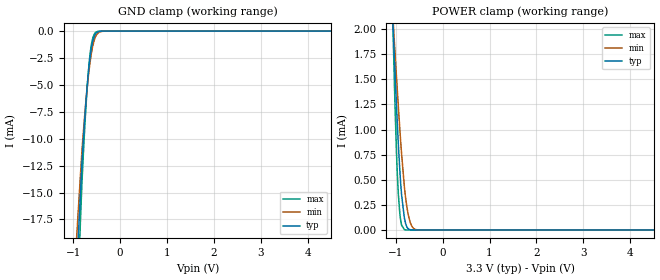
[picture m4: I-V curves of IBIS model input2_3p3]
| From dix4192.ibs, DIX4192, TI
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|   input2_3p3 Model
[Model]   input2_3p3
Model_type   Input
Vinl = 0.99
Vinh = 2.31
|   typ   min   max
C_comp   30.3138pF   24.4141pF   36.1111pF
[Model spec]
|subparameter
Vinl   0.99   0.90   1.08
Vinh   2.31   2.10   2.52
| Where nom  PVT is Nominal Process, 3.3V, 27C
|   Fast PVT is Strong Process,  3.6V, -40C
|   Slow PVT is Weak Process,   3.0V, 105C
[Voltage Range]   3.3   3   3.6
[Temperature Range]   27   105   -40
[Power Clamp Reference]   3.3   3   3.6
[GND Clamp Reference]   0   0   0
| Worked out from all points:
|   GND clamp passes 1 mA (typ) near -0.59 V on its own axis
|   POWER clamp passes 1 mA (typ) near -0.96 V on its own axis
[GND Clamp]
|   Voltage   I(typ)   I(min)   I(max)
-3.3V     -1.038A    -961.1mA   -1.11A
-1.142V   -41.66mA   -34.56mA   -50.89mA
-815.1mV  -12.29mA   -11.2mA    -14.22mA
-765.6mV  -8.848mA   -8.391mA   -9.888mA
-726mV    -6.414mA   -6.372mA   -6.859mA
-686.4mV  -4.331mA   -4.594mA   -4.322mA
-656.7mV  -3.038mA   -3.444mA   -2.811mA
-627mV    -2.016mA   -2.471mA   -1.672mA
-587.4mV  -1.024mA   -1.467mA   -717.4uA
-498.3mV  -142.2uA   -317uA     -60.17uA
-260.7mV  0A         -706.3nA   0A
6.6V      0A         0A         0A
[POWER Clamp]
|   Voltage   I(typ)   I(min)   I(max)
-3.3V     31.5mA     22.11mA    54.06mA
-1.063V   2.111mA    2.146mA    2.099mA
-1.053V   1.997mA    2.066mA    1.911mA
-1.013V   1.555mA    1.753mA    1.213mA
-983.4mV  1.24mA     1.524mA    773.4uA
-943.8mV  854.9uA    1.228mA    359.1uA
-894.3mV  464.9uA    884uA      96.47uA
-815.1mV  120.1uA    431uA      3.519uA
-755.7mV  25.1uA     212uA      70.9nA
-696.3mV  3.16uA     85.49uA    0A
-547.8mV  0A         1.94uA     0A
6.6V      0A         0A         0A
